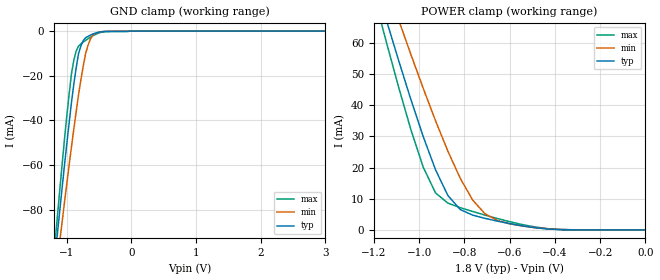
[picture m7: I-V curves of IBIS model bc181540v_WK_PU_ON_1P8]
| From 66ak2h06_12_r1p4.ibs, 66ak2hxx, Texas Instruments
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|   Model Cell bc181540v_WK_PU_ON_1P8
|bc181540v_WK_PU_ON_1P8
[Model]   bc181540v_WK_PU_ON_1P8
Model_type   Input
Polarity   Non-Inverting
Vinl =  0.63
Vinh =  1.17
C_comp   1.16613p   0.553312p   1.16742p
[Model Spec]
Vinl   0.63   0.567   0.693
Vinh   1.17   1.053   1.287
[Temperature Range]   25   125   -40
[Voltage Range]   1.8   1.62   1.98
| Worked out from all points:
|   GND clamp passes 1 mA (typ) near -0.57 V on its own axis
|   POWER clamp passes 1 mA (typ) near -0.51 V on its own axis
[POWER_clamp]
|   voltage   I(typ)   I(min)   I(max)
-1.8V     235.9mA    223mA      250.8mA
-1.164V   71.91mA    82.68mA    65.42mA
-1.127V   63.11mA    75.02mA    55.57mA
-1.073V   50.21mA    63.7mA     41.31mA
-981.8mV  29.92mA    45.39mA    20.13mA
-927.3mV  19.27mA    34.97mA    11.86mA
-872.7mV  11.04mA    25.23mA    8.599mA
-818.2mV  6.545mA    16.55mA    7.145mA
-763.6mV  4.758mA    9.631mA    5.926mA
-709.1mV  3.717mA    5.192mA    4.769mA
-490.9mV  745.5uA    782.8uA    994.9uA
0V        968.3pA    18.35nA    2.392nA
[GND_clamp]
|   voltage   I(typ)   I(min)   I(max)
-1.8V     -286.5mA   -268.3mA   -306.4mA
-1.182V   -101.6mA   -112.2mA   -95.23mA
-1.145V   -91.07mA   -103.3mA   -83.3mA
-1.109V   -80.75mA   -94.49mA   -71.63mA
-1.073V   -70.54mA   -85.75mA   -60.14mA
-963.6mV  -41.22mA   -60.16mA   -28.35mA
-890.9mV  -23.79mA   -43.89mA   -13.12mA
-818.2mV  -10.12mA   -28.64mA   -6.746mA
-672.7mV  -2.372mA   -6.469mA   -3.459mA
-600mV    -1.342mA   -1.913mA   -2.146mA
-418.2mV  -198.9uA   -162.5uA   -336.4uA
3.6V      0A         0A         0A
